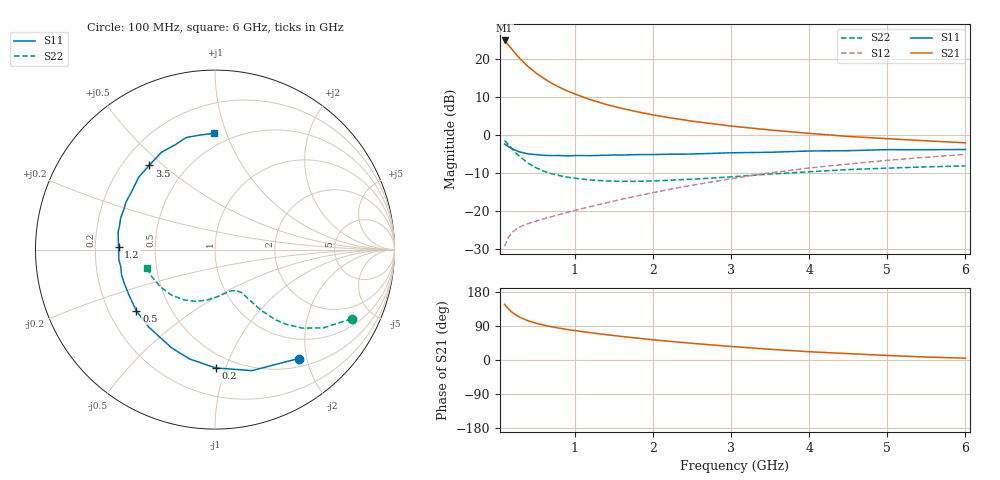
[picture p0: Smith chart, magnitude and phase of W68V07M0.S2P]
! SIEMENS Small Signal Semiconductors
! BFR193W
! Si NPN RF Bipolar Junction Transistor in SOT323
! VCE = 8 V  IC = 7 mA
! Common Emitter S-Parameters:  September  1992
# GHz  S  MA  R  50
!  f  S11  S21  S12  S22
! GHz  MAG  ANG  MAG  ANG  MAG  ANG  MAG  ANG
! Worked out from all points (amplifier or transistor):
!   28 points, 100 MHz to 6 GHz, reference 50 ohm
!   highest |S21| = 24.9 dB at 100 MHz (marker M1)
!   |S21| within 3 dB of that: start of sweep to 221.6 MHz
!   unconditionally stable (mu >= 1): 1.137 GHz to 2.602 GHz
!   at 300 MHz: K = 0.44, MSG = 22.1 dB, |S12| = -24.1 dB
!   at 1.5 GHz: K = 1.05, MAG = 11.1 dB, |S12| = -17.3 dB
!   at 6 GHz: K = 0.88, MSG = 1.5 dB, |S12| = -5.1 dB
!   lowest NFmin = 1.20 dB at 450 MHz
!   S11 on the Smith chart (normalised r, x): 100 MHz: 0.63, -1.86; 200 MHz: 0.40, -0.92; 500 MHz: 0.32, -0.31; 1.2 GHz: 0.30, +0.01; 3.5 GHz: 0.31, +0.45; 6 GHz: 0.41, +0.90
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0.1  0.765 -52.5  17.57 146.9  0.0347 65.0  0.8528 -26.9
0.15  0.7049 -73.1  15.26 134.6  0.0456 57.3  0.7464 -35.7
0.2  0.6592 -89.7  13.22 125.2  0.0529 51.9  0.6539 -42.0
0.25  0.6257 -103.0  11.47 118.1  0.0583 48.8  0.5747 -46.4
0.3  0.5989 -113.7  10.07 112.3  0.0624 46.8  0.5165 -49.2
0.4  0.5681 -130.6  7.988 103.6  0.0686 45.6  0.4289 -52.6
0.5  0.5552 -142.1  6.586 97.3  0.0739 46.1  0.3737 -54.3
0.6  0.5429 -151.2  5.589 92.2  0.0796 47.2  0.3363 -55.8
0.7  0.5392 -158.4  4.827 87.8  0.0847 48.8  0.3117 -56.6
0.8  0.5396 -164.6  4.273 84.0  0.0901 50.6  0.2938 -57.8
0.9  0.5336 -169.7  3.82 80.6  0.0962 52.2  0.2803 -58.5
1  0.5386 -173.9  3.474 77.5  0.1023 53.7  0.2718 -59.8
1.2  0.5378 178.3  2.923 72.0  0.1151 56.1  0.2571 -62.7
1.4  0.5443 172.1  2.534 66.9  0.1288 58.3  0.2502 -65.9
1.6  0.5478 166.6  2.249 62.1  0.1437 59.8  0.2467 -69.3
1.8  0.5544 161.6  2.026 57.7  0.1593 61.0  0.2469 -73.4
2.2  0.5619 152.1  1.7 49.6  0.1926 62.1  0.2545 -81.2
3  0.5865 136.4  1.317 35.7  0.2674 60.9  0.2827 -98.2
3.5  0.5953 128.0  1.169 28.3  0.3198 58.1  0.3082 -110.4
4.5  0.6246 110.8  0.962 16.8  0.417 50.2  0.3526 -134.6
5.5  0.6436 97.5  0.842 7.8  0.5129 41.4  0.3824 -156.4
6  0.6476 90.6  0.793 4.7  0.5587 36.2  0.394 -164.6
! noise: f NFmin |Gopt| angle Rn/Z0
0.45  1.2  0.24  125  0.12
0.9  1.25  0.36  154  0.11
1.8  2  0.55  -156  0.13
